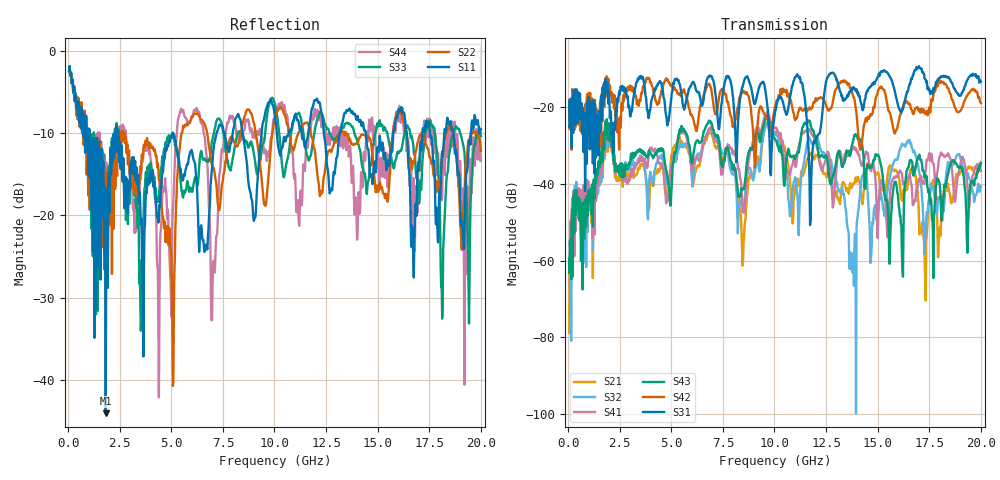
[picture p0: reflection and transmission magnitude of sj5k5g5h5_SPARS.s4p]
! FILE: E:\users\goganessyan\GBX_Backplane\FR408_backplane\1m_OUTBOUND_NEXT\sj5k5g5h5_SPARS.s4p
# MHZ S RI R 50.00
! FREQ  S11  S12  S13  S14
!  S21  S22  S23  S24
!  S31  S32  S33  S34
!  S41  S42  S43  S44
!  REAL  IMAG  REAL  IMAG  REAL  IMAG  REAL  IMAG
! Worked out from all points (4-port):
!   799 points, 50 MHz to 20 GHz, reference 50 ohm
!   strongest paths, dB at 50 MHz, 5.025 GHz, 10.03 GHz, 15.03 GHz, 20 GHz:
!     S31: -18.6, -16.3, -21.4, -12.1, -13.4
!     S42: -18.2, -14.7, -20.0, -15.6, -19.0
!     S43: -59.4, -40.2, -28.3, -32.4, -34.7
!     S41: -59.4, -35.1, -25.3, -49.6, -36.7
!     S32: -55.1, -34.6, -26.6, -46.9, -40.8
!     S21: -60.8, -32.2, -26.6, -37.1, -34.3
!   lowest |S11| = -44.1 dB at 1.825 GHz (marker M1), VSWR 1.01, Z = 50.6 + j0.0386 ohm
!   |S11| at or under -10 dB: 2.433 GHz to 5.063 GHz (2.63 GHz wide, 70.2 % of centre); 5.078 GHz to 7.201 GHz (2.123 GHz wide, 34.6 % of centre); 14.43 GHz to 15.75 GHz (1.323 GHz wide, 8.77 % of centre)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
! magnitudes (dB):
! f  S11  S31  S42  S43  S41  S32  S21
! 50 MHz  -2.5  -18.6  -18.2  -59.4  -59.4  -55.1  -60.8
! 1.825 GHz  -44.1  -12.7  -17.3  -26.7  -27.5  -28.0  -28.8
! 11.15 GHz  -8.5  -11.9  -21.4  -31.7  -30.7  -48.0  -39.5
! 11.75 GHz  -8.1  -49.4  -20.7  -24.8  -26.6  -28.7  -32.2
! 13.78 GHz  -7.4  -15.5  -16.5  -29.6  -30.8  -63.1  -40.6
! 16.48 GHz  -13.3  -15.7  -19.0  -35.7  -38.6  -29.3  -39.5
! 20 GHz  -9.6  -13.4  -19.0  -34.7  -36.7  -40.8  -34.3
